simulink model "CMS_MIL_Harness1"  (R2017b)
settings: Solver=FixedStepDiscrete  StartTime=0.0  StopTime=23  FixedStep=0.01  RelTol=1e-3  EnableMultiTasking=on
undefined symbols (not defined in the file): sigbuilder_block
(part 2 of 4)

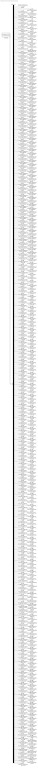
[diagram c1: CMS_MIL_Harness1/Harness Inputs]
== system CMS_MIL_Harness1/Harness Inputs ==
  Demux : Demux  Tag=STV Demux  Outputs=413
  FromWs : FromWorkspace  Tag=STV FromWs  VariableName=tuvar  SampleTime=0
  GeCTC_CtrCtlState_enum : Outport  Tag=STV Outport
  GbCTC_NegCtlState_flg : Outport  Tag=STV Outport  Port=2
  GbCTC_PosCtlState_flg : Outport  Tag=STV Outport  Port=3
  GbCTC_DCPosChrgCtlState_flg : Outport  Tag=STV Outport  Port=4
  GbCTC_DCNegChrgCtlState_flg : Outport  Tag=STV Outport  Port=5
  GcHDP_PackVolt_V : Outport  Tag=STV Outport  Port=6
  GbCTC_PreChrgCtlState_flg : Outport  Tag=STV Outport  Port=7
  GcHDP_PackCrnt_A : Outport  Tag=STV Outport  Port=8
  GbWSM_Kl15WkUpPrs_flg : Outport  Tag=STV Outport  Port=9
  GcCDP_MinCellVolt_mV : Outport  Tag=STV Outport  Port=10
  GcCDP_MaxCellVolt_mV : Outport  Tag=STV Outport  Port=11
  GbACC_ObcChrgCmd_flg : Outport  Tag=STV Outport  Port=12
  GcACC_ACChrgVoltRqst_V : Outport  Tag=STV Outport  Port=13
  GcACC_ACChrgCrntRqst_A : Outport  Tag=STV Outport  Port=14
  GbACC_ACChrgRqst_flg : Outport  Tag=STV Outport  Port=15
  GeCTC_CtrCtlConnMode_enum : Outport  Tag=STV Outport  Port=16
  GbMSM_SelfCheck_flg : Outport  Tag=STV Outport  Port=17
  GcSOC_DispSOC_pct : Outport  Tag=STV Outport  Port=18
  GbISP_TFHvilLFlt_flg : Outport  Tag=STV Outport  Port=19
  GeFTC_FltLvlOnCAN_enum : Outport  Tag=STV Outport  Port=20
  GcSOH_PackSOH_pct : Outport  Tag=STV Outport  Port=21
  GcSOC_PackSOC_pct : Outport  Tag=STV Outport  Port=22
  GcHDP_HallCrnt_A : Outport  Tag=STV Outport  Port=23
  GbMSM_SelfChckMaxTiReach_flg : Outport  Tag=STV Outport  Port=24
  GaCBC_CellBalCtlCmd_flg(1) : Outport  Tag=STV Outport  Port=25
  GaCBC_CellBalCtlCmd_flg(2) : Outport  Tag=STV Outport  Port=26
  GaCBC_CellBalCtlCmd_flg(3) : Outport  Tag=STV Outport  Port=27
  GaCBC_CellBalCtlCmd_flg(4) : Outport  Tag=STV Outport  Port=28
  GaCBC_CellBalCtlCmd_flg(5) : Outport  Tag=STV Outport  Port=29
  GaCBC_CellBalCtlCmd_flg(6) : Outport  Tag=STV Outport  Port=30
  GaCBC_CellBalCtlCmd_flg(7) : Outport  Tag=STV Outport  Port=31
  GaCBC_CellBalCtlCmd_flg(8) : Outport  Tag=STV Outport  Port=32
  GaCBC_CellBalCtlCmd_flg(9) : Outport  Tag=STV Outport  Port=33
  GaCBC_CellBalCtlCmd_flg(10) : Outport  Tag=STV Outport  Port=34
  GaCBC_CellBalCtlCmd_flg(11) : Outport  Tag=STV Outport  Port=35
  GaCBC_CellBalCtlCmd_flg(12) : Outport  Tag=STV Outport  Port=36
  GaCBC_CellBalCtlCmd_flg(13) : Outport  Tag=STV Outport  Port=37
  GaCBC_CellBalCtlCmd_flg(14) : Outport  Tag=STV Outport  Port=38
  GaCBC_CellBalCtlCmd_flg(15) : Outport  Tag=STV Outport  Port=39
  GaCBC_CellBalCtlCmd_flg(16) : Outport  Tag=STV Outport  Port=40
  GaCBC_CellBalCtlCmd_flg(17) : Outport  Tag=STV Outport  Port=41
  GaCBC_CellBalCtlCmd_flg(18) : Outport  Tag=STV Outport  Port=42
  GaCBC_CellBalCtlCmd_flg(19) : Outport  Tag=STV Outport  Port=43
  GaCBC_CellBalCtlCmd_flg(20) : Outport  Tag=STV Outport  Port=44
  GaCBC_CellBalCtlCmd_flg(21) : Outport  Tag=STV Outport  Port=45
  GaCBC_CellBalCtlCmd_flg(22) : Outport  Tag=STV Outport  Port=46
  GaCBC_CellBalCtlCmd_flg(23) : Outport  Tag=STV Outport  Port=47
  GaCBC_CellBalCtlCmd_flg(24) : Outport  Tag=STV Outport  Port=48
  GaCBC_CellBalCtlCmd_flg(25) : Outport  Tag=STV Outport  Port=49
  GaCBC_CellBalCtlCmd_flg(26) : Outport  Tag=STV Outport  Port=50
  GaCBC_CellBalCtlCmd_flg(27) : Outport  Tag=STV Outport  Port=51
  GaCBC_CellBalCtlCmd_flg(28) : Outport  Tag=STV Outport  Port=52
  GaCBC_CellBalCtlCmd_flg(29) : Outport  Tag=STV Outport  Port=53
  GaCBC_CellBalCtlCmd_flg(30) : Outport  Tag=STV Outport  Port=54
  GaCBC_CellBalCtlCmd_flg(31) : Outport  Tag=STV Outport  Port=55
  GaCBC_CellBalCtlCmd_flg(32) : Outport  Tag=STV Outport  Port=56
  GaCBC_CellBalCtlCmd_flg(33) : Outport  Tag=STV Outport  Port=57
  GaCBC_CellBalCtlCmd_flg(34) : Outport  Tag=STV Outport  Port=58
  GaCBC_CellBalCtlCmd_flg(35) : Outport  Tag=STV Outport  Port=59
  GaCBC_CellBalCtlCmd_flg(36) : Outport  Tag=STV Outport  Port=60
  GaCBC_CellBalCtlCmd_flg(37) : Outport  Tag=STV Outport  Port=61
  GaCBC_CellBalCtlCmd_flg(38) : Outport  Tag=STV Outport  Port=62
  GaCBC_CellBalCtlCmd_flg(39) : Outport  Tag=STV Outport  Port=63
  GaCBC_CellBalCtlCmd_flg(40) : Outport  Tag=STV Outport  Port=64
  GaCBC_CellBalCtlCmd_flg(41) : Outport  Tag=STV Outport  Port=65
  GaCBC_CellBalCtlCmd_flg(42) : Outport  Tag=STV Outport  Port=66
  GaCBC_CellBalCtlCmd_flg(43) : Outport  Tag=STV Outport  Port=67
  GaCBC_CellBalCtlCmd_flg(44) : Outport  Tag=STV Outport  Port=68
  GaCBC_CellBalCtlCmd_flg(45) : Outport  Tag=STV Outport  Port=69
  GaCBC_CellBalCtlCmd_flg(46) : Outport  Tag=STV Outport  Port=70
  GaCBC_CellBalCtlCmd_flg(47) : Outport  Tag=STV Outport  Port=71
  GaCBC_CellBalCtlCmd_flg(48) : Outport  Tag=STV Outport  Port=72
  GaCBC_CellBalCtlCmd_flg(49) : Outport  Tag=STV Outport  Port=73
  GaCBC_CellBalCtlCmd_flg(50) : Outport  Tag=STV Outport  Port=74
  GaCBC_CellBalCtlCmd_flg(51) : Outport  Tag=STV Outport  Port=75
  GaCBC_CellBalCtlCmd_flg(52) : Outport  Tag=STV Outport  Port=76
  GaCBC_CellBalCtlCmd_flg(53) : Outport  Tag=STV Outport  Port=77
  GaCBC_CellBalCtlCmd_flg(54) : Outport  Tag=STV Outport  Port=78
  GaCBC_CellBalCtlCmd_flg(55) : Outport  Tag=STV Outport  Port=79
  GaCBC_CellBalCtlCmd_flg(56) : Outport  Tag=STV Outport  Port=80
  GaCBC_CellBalCtlCmd_flg(57) : Outport  Tag=STV Outport  Port=81
  GaCBC_CellBalCtlCmd_flg(58) : Outport  Tag=STV Outport  Port=82
  GaCBC_CellBalCtlCmd_flg(59) : Outport  Tag=STV Outport  Port=83
  GaCBC_CellBalCtlCmd_flg(60) : Outport  Tag=STV Outport  Port=84
  GaCBC_CellBalCtlCmd_flg(61) : Outport  Tag=STV Outport  Port=85
  GaCBC_CellBalCtlCmd_flg(62) : Outport  Tag=STV Outport  Port=86
  GaCBC_CellBalCtlCmd_flg(63) : Outport  Tag=STV Outport  Port=87
  GaCBC_CellBalCtlCmd_flg(64) : Outport  Tag=STV Outport  Port=88
  GaCBC_CellBalCtlCmd_flg(65) : Outport  Tag=STV Outport  Port=89
  GaCBC_CellBalCtlCmd_flg(66) : Outport  Tag=STV Outport  Port=90
  GaCBC_CellBalCtlCmd_flg(67) : Outport  Tag=STV Outport  Port=91
  GaCBC_CellBalCtlCmd_flg(68) : Outport  Tag=STV Outport  Port=92
  GaCBC_CellBalCtlCmd_flg(69) : Outport  Tag=STV Outport  Port=93
  GaCBC_CellBalCtlCmd_flg(70) : Outport  Tag=STV Outport  Port=94
  GaCBC_CellBalCtlCmd_flg(71) : Outport  Tag=STV Outport  Port=95
  GaCBC_CellBalCtlCmd_flg(72) : Outport  Tag=STV Outport  Port=96
  GaCBC_CellBalCtlCmd_flg(73) : Outport  Tag=STV Outport  Port=97
  GaCBC_CellBalCtlCmd_flg(74) : Outport  Tag=STV Outport  Port=98
  GaCBC_CellBalCtlCmd_flg(75) : Outport  Tag=STV Outport  Port=99
  GaCBC_CellBalCtlCmd_flg(76) : Outport  Tag=STV Outport  Port=100
  GaCBC_CellBalCtlCmd_flg(77) : Outport  Tag=STV Outport  Port=101
  GaCBC_CellBalCtlCmd_flg(78) : Outport  Tag=STV Outport  Port=102
  GaCBC_CellBalCtlCmd_flg(79) : Outport  Tag=STV Outport  Port=103
  GaCBC_CellBalCtlCmd_flg(80) : Outport  Tag=STV Outport  Port=104
  GaCBC_CellBalCtlCmd_flg(81) : Outport  Tag=STV Outport  Port=105
  GaCBC_CellBalCtlCmd_flg(82) : Outport  Tag=STV Outport  Port=106
  GaCBC_CellBalCtlCmd_flg(83) : Outport  Tag=STV Outport  Port=107
  GaCBC_CellBalCtlCmd_flg(84) : Outport  Tag=STV Outport  Port=108
  GaCBC_CellBalCtlCmd_flg(85) : Outport  Tag=STV Outport  Port=109
  GaCBC_CellBalCtlCmd_flg(86) : Outport  Tag=STV Outport  Port=110
  GaCBC_CellBalCtlCmd_flg(87) : Outport  Tag=STV Outport  Port=111
  GaCBC_CellBalCtlCmd_flg(88) : Outport  Tag=STV Outport  Port=112
  GaCBC_CellBalCtlCmd_flg(89) : Outport  Tag=STV Outport  Port=113
  GaCBC_CellBalCtlCmd_flg(90) : Outport  Tag=STV Outport  Port=114
  GaCBC_CellBalCtlCmd_flg(91) : Outport  Tag=STV Outport  Port=115
  GaCBC_CellBalCtlCmd_flg(92) : Outport  Tag=STV Outport  Port=116
  GaCBC_CellBalCtlCmd_flg(93) : Outport  Tag=STV Outport  Port=117
  GaCBC_CellBalCtlCmd_flg(94) : Outport  Tag=STV Outport  Port=118
  GaCBC_CellBalCtlCmd_flg(95) : Outport  Tag=STV Outport  Port=119
  GaCBC_CellBalCtlCmd_flg(96) : Outport  Tag=STV Outport  Port=120
  GaCBC_CellBalCtlCmd_flg(97) : Outport  Tag=STV Outport  Port=121
  GaCBC_CellBalCtlCmd_flg(98) : Outport  Tag=STV Outport  Port=122
  GaCBC_CellBalCtlCmd_flg(99) : Outport  Tag=STV Outport  Port=123
  GaCBC_CellBalCtlCmd_flg(100) : Outport  Tag=STV Outport  Port=124
  GaCBC_CellBalCtlCmd_flg(101) : Outport  Tag=STV Outport  Port=125
  GaCBC_CellBalCtlCmd_flg(102) : Outport  Tag=STV Outport  Port=126
  GaCBC_CellBalCtlCmd_flg(103) : Outport  Tag=STV Outport  Port=127
  GaCBC_CellBalCtlCmd_flg(104) : Outport  Tag=STV Outport  Port=128
  GaCBC_CellBalCtlCmd_flg(105) : Outport  Tag=STV Outport  Port=129
  GaCBC_CellBalCtlCmd_flg(106) : Outport  Tag=STV Outport  Port=130
  GaCBC_CellBalCtlCmd_flg(107) : Outport  Tag=STV Outport  Port=131
  GaCBC_CellBalCtlCmd_flg(108) : Outport  Tag=STV Outport  Port=132
  GaCBC_CellBalCtlCmd_flg(109) : Outport  Tag=STV Outport  Port=133
  GaCBC_CellBalCtlCmd_flg(110) : Outport  Tag=STV Outport  Port=134
  GaCBC_CellBalCtlCmd_flg(111) : Outport  Tag=STV Outport  Port=135
  GaCBC_CellBalCtlCmd_flg(112) : Outport  Tag=STV Outport  Port=136
  GbDCC_DCChrgRqst_flg : Outport  Tag=STV Outport  Port=137
  GcSOP_DischrgConstPwr_kW : Outport  Tag=STV Outport  Port=138
  GcSOP_ChrgConstPwr_kW : Outport  Tag=STV Outport  Port=139
  GcISO_HVIsoValue_kohm : Outport  Tag=STV Outport  Port=140
  GeODP_ObcCcSt_enum : Outport  Tag=STV Outport  Port=141
  GbDCC_DCChrgFinish_flg : Outport  Tag=STV Outport  Port=142
  GbACC_ACChrgFinish_flg : Outport  Tag=STV Outport  Port=143
  GeACC_ACChrgState_enum : Outport  Tag=STV Outport  Port=144
  GeDCC_DCConnSt_enum : Outport  Tag=STV Outport  Port=145
  GeLDP_CC2St_enum : Outport  Tag=STV Outport  Port=146
  GcCDP_AvgCellTemp_C : Outport  Tag=STV Outport  Port=147
  GbISO_IsoForbid_flg : Outport  Tag=STV Outport  Port=148
  GcCDP_MaxCellTemp_C : Outport  Tag=STV Outport  Port=149
  GcCDP_MinCellTemp_C : Outport  Tag=STV Outport  Port=150
  GcDCS_3072ChrgVoltReq_V : Outport  Tag=STV Outport  Port=151
  GcDCC_DCChrgCrntRqst_A : Outport  Tag=STV Outport  Port=152
  GaCDP_CellVolt_mV(1) : Outport  Tag=STV Outport  Port=153
  GaCDP_CellVolt_mV(2) : Outport  Tag=STV Outport  Port=154
  GaCDP_CellVolt_mV(3) : Outport  Tag=STV Outport  Port=155
  GaCDP_CellVolt_mV(4) : Outport  Tag=STV Outport  Port=156
  GaCDP_CellVolt_mV(5) : Outport  Tag=STV Outport  Port=157
  GaCDP_CellVolt_mV(6) : Outport  Tag=STV Outport  Port=158
  GaCDP_CellVolt_mV(7) : Outport  Tag=STV Outport  Port=159
  GaCDP_CellVolt_mV(8) : Outport  Tag=STV Outport  Port=160
  GaCDP_CellVolt_mV(9) : Outport  Tag=STV Outport  Port=161
  GaCDP_CellVolt_mV(10) : Outport  Tag=STV Outport  Port=162
  GaCDP_CellVolt_mV(11) : Outport  Tag=STV Outport  Port=163
  GaCDP_CellVolt_mV(12) : Outport  Tag=STV Outport  Port=164
  GaCDP_CellVolt_mV(13) : Outport  Tag=STV Outport  Port=165
  GaCDP_CellVolt_mV(14) : Outport  Tag=STV Outport  Port=166
  GaCDP_CellVolt_mV(15) : Outport  Tag=STV Outport  Port=167
  GaCDP_CellVolt_mV(16) : Outport  Tag=STV Outport  Port=168
  GaCDP_CellVolt_mV(17) : Outport  Tag=STV Outport  Port=169
  GaCDP_CellVolt_mV(18) : Outport  Tag=STV Outport  Port=170
  GaCDP_CellVolt_mV(19) : Outport  Tag=STV Outport  Port=171
  GaCDP_CellVolt_mV(20) : Outport  Tag=STV Outport  Port=172
  GaCDP_CellVolt_mV(21) : Outport  Tag=STV Outport  Port=173
  GaCDP_CellVolt_mV(22) : Outport  Tag=STV Outport  Port=174
  GaCDP_CellVolt_mV(23) : Outport  Tag=STV Outport  Port=175
  GaCDP_CellVolt_mV(24) : Outport  Tag=STV Outport  Port=176
  GaCDP_CellVolt_mV(25) : Outport  Tag=STV Outport  Port=177
  GaCDP_CellVolt_mV(26) : Outport  Tag=STV Outport  Port=178
  GaCDP_CellVolt_mV(27) : Outport  Tag=STV Outport  Port=179
  GaCDP_CellVolt_mV(28) : Outport  Tag=STV Outport  Port=180
  GaCDP_CellVolt_mV(29) : Outport  Tag=STV Outport  Port=181
  GaCDP_CellVolt_mV(30) : Outport  Tag=STV Outport  Port=182
  GaCDP_CellVolt_mV(31) : Outport  Tag=STV Outport  Port=183
  GaCDP_CellVolt_mV(32) : Outport  Tag=STV Outport  Port=184
  GaCDP_CellVolt_mV(33) : Outport  Tag=STV Outport  Port=185
  GaCDP_CellVolt_mV(34) : Outport  Tag=STV Outport  Port=186
  GaCDP_CellVolt_mV(35) : Outport  Tag=STV Outport  Port=187
  GaCDP_CellVolt_mV(36) : Outport  Tag=STV Outport  Port=188
  GaCDP_CellVolt_mV(37) : Outport  Tag=STV Outport  Port=189
  GaCDP_CellVolt_mV(38) : Outport  Tag=STV Outport  Port=190
  GaCDP_CellVolt_mV(39) : Outport  Tag=STV Outport  Port=191
  GaCDP_CellVolt_mV(40) : Outport  Tag=STV Outport  Port=192
  GaCDP_CellVolt_mV(41) : Outport  Tag=STV Outport  Port=193
  GaCDP_CellVolt_mV(42) : Outport  Tag=STV Outport  Port=194
  GaCDP_CellVolt_mV(43) : Outport  Tag=STV Outport  Port=195
  GaCDP_CellVolt_mV(44) : Outport  Tag=STV Outport  Port=196
  GaCDP_CellVolt_mV(45) : Outport  Tag=STV Outport  Port=197
  GaCDP_CellVolt_mV(46) : Outport  Tag=STV Outport  Port=198
  GaCDP_CellVolt_mV(47) : Outport  Tag=STV Outport  Port=199
  GaCDP_CellVolt_mV(48) : Outport  Tag=STV Outport  Port=200
  GaCDP_CellVolt_mV(49) : Outport  Tag=STV Outport  Port=201
  GaCDP_CellVolt_mV(50) : Outport  Tag=STV Outport  Port=202
  GaCDP_CellVolt_mV(51) : Outport  Tag=STV Outport  Port=203
  GaCDP_CellVolt_mV(52) : Outport  Tag=STV Outport  Port=204
  GaCDP_CellVolt_mV(53) : Outport  Tag=STV Outport  Port=205
  GaCDP_CellVolt_mV(54) : Outport  Tag=STV Outport  Port=206
  GaCDP_CellVolt_mV(55) : Outport  Tag=STV Outport  Port=207
  GaCDP_CellVolt_mV(56) : Outport  Tag=STV Outport  Port=208
  GaCDP_CellVolt_mV(57) : Outport  Tag=STV Outport  Port=209
  GaCDP_CellVolt_mV(58) : Outport  Tag=STV Outport  Port=210
  GaCDP_CellVolt_mV(59) : Outport  Tag=STV Outport  Port=211
  GaCDP_CellVolt_mV(60) : Outport  Tag=STV Outport  Port=212
  GaCDP_CellVolt_mV(61) : Outport  Tag=STV Outport  Port=213
  GaCDP_CellVolt_mV(62) : Outport  Tag=STV Outport  Port=214
  GaCDP_CellVolt_mV(63) : Outport  Tag=STV Outport  Port=215
  GaCDP_CellVolt_mV(64) : Outport  Tag=STV Outport  Port=216
  GaCDP_CellVolt_mV(65) : Outport  Tag=STV Outport  Port=217
  GaCDP_CellVolt_mV(66) : Outport  Tag=STV Outport  Port=218
  GaCDP_CellVolt_mV(67) : Outport  Tag=STV Outport  Port=219
  GaCDP_CellVolt_mV(68) : Outport  Tag=STV Outport  Port=220
  GaCDP_CellVolt_mV(69) : Outport  Tag=STV Outport  Port=221
  GaCDP_CellVolt_mV(70) : Outport  Tag=STV Outport  Port=222
  GaCDP_CellVolt_mV(71) : Outport  Tag=STV Outport  Port=223
  GaCDP_CellVolt_mV(72) : Outport  Tag=STV Outport  Port=224
  GaCDP_CellVolt_mV(73) : Outport  Tag=STV Outport  Port=225
  GaCDP_CellVolt_mV(74) : Outport  Tag=STV Outport  Port=226
  GaCDP_CellVolt_mV(75) : Outport  Tag=STV Outport  Port=227
  GaCDP_CellVolt_mV(76) : Outport  Tag=STV Outport  Port=228
  GaCDP_CellVolt_mV(77) : Outport  Tag=STV Outport  Port=229
  GaCDP_CellVolt_mV(78) : Outport  Tag=STV Outport  Port=230
  GaCDP_CellVolt_mV(79) : Outport  Tag=STV Outport  Port=231
  GaCDP_CellVolt_mV(80) : Outport  Tag=STV Outport  Port=232
  GaCDP_CellVolt_mV(81) : Outport  Tag=STV Outport  Port=233
  GaCDP_CellVolt_mV(82) : Outport  Tag=STV Outport  Port=234
  GaCDP_CellVolt_mV(83) : Outport  Tag=STV Outport  Port=235
  GaCDP_CellVolt_mV(84) : Outport  Tag=STV Outport  Port=236
  GaCDP_CellVolt_mV(85) : Outport  Tag=STV Outport  Port=237
  GaCDP_CellVolt_mV(86) : Outport  Tag=STV Outport  Port=238
  GaCDP_CellVolt_mV(87) : Outport  Tag=STV Outport  Port=239
  GaCDP_CellVolt_mV(88) : Outport  Tag=STV Outport  Port=240
  GaCDP_CellVolt_mV(89) : Outport  Tag=STV Outport  Port=241
  GaCDP_CellVolt_mV(90) : Outport  Tag=STV Outport  Port=242
  GaCDP_CellVolt_mV(91) : Outport  Tag=STV Outport  Port=243
  GaCDP_CellVolt_mV(92) : Outport  Tag=STV Outport  Port=244
  GaCDP_CellVolt_mV(93) : Outport  Tag=STV Outport  Port=245
  GaCDP_CellVolt_mV(94) : Outport  Tag=STV Outport  Port=246
  GaCDP_CellVolt_mV(95) : Outport  Tag=STV Outport  Port=247
  GaCDP_CellVolt_mV(96) : Outport  Tag=STV Outport  Port=248
  GaCDP_CellVolt_mV(97) : Outport  Tag=STV Outport  Port=249
  GaCDP_CellVolt_mV(98) : Outport  Tag=STV Outport  Port=250
  GaCDP_CellVolt_mV(99) : Outport  Tag=STV Outport  Port=251
  GaCDP_CellVolt_mV(100) : Outport  Tag=STV Outport  Port=252
  GaCDP_CellVolt_mV(101) : Outport  Tag=STV Outport  Port=253
  GaCDP_CellVolt_mV(102) : Outport  Tag=STV Outport  Port=254
  GaCDP_CellVolt_mV(103) : Outport  Tag=STV Outport  Port=255
  GaCDP_CellVolt_mV(104) : Outport  Tag=STV Outport  Port=256
  GaCDP_CellVolt_mV(105) : Outport  Tag=STV Outport  Port=257
  GaCDP_CellVolt_mV(106) : Outport  Tag=STV Outport  Port=258
  GaCDP_CellVolt_mV(107) : Outport  Tag=STV Outport  Port=259
  GaCDP_CellVolt_mV(108) : Outport  Tag=STV Outport  Port=260
  GaCDP_CellVolt_mV(109) : Outport  Tag=STV Outport  Port=261
  GaCDP_CellVolt_mV(110) : Outport  Tag=STV Outport  Port=262
  GaCDP_CellVolt_mV(111) : Outport  Tag=STV Outport  Port=263
  GaCDP_CellVolt_mV(112) : Outport  Tag=STV Outport  Port=264
  GaCDP_CellTemp_C(1) : Outport  Tag=STV Outport  Port=265
  GaCDP_CellTemp_C(2) : Outport  Tag=STV Outport  Port=266
  GaCDP_CellTemp_C(3) : Outport  Tag=STV Outport  Port=267
  GaCDP_CellTemp_C(4) : Outport  Tag=STV Outport  Port=268
  GaCDP_CellTemp_C(5) : Outport  Tag=STV Outport  Port=269
  GaCDP_CellTemp_C(6) : Outport  Tag=STV Outport  Port=270
  GaCDP_CellTemp_C(7) : Outport  Tag=STV Outport  Port=271
  GaCDP_CellTemp_C(8) : Outport  Tag=STV Outport  Port=272
  GaCDP_CellTemp_C(9) : Outport  Tag=STV Outport  Port=273
  GaCDP_CellTemp_C(10) : Outport  Tag=STV Outport  Port=274
  GaCDP_CellTemp_C(11) : Outport  Tag=STV Outport  Port=275
  GaCDP_CellTemp_C(12) : Outport  Tag=STV Outport  Port=276
  GaCDP_CellTemp_C(13) : Outport  Tag=STV Outport  Port=277
  GaCDP_CellTemp_C(14) : Outport  Tag=STV Outport  Port=278
  GaCDP_CellTemp_C(15) : Outport  Tag=STV Outport  Port=279
  GaCDP_CellTemp_C(16) : Outport  Tag=STV Outport  Port=280
  GaCDP_CellTemp_C(17) : Outport  Tag=STV Outport  Port=281
  GaCDP_CellTemp_C(18) : Outport  Tag=STV Outport  Port=282
  GaCDP_CellTemp_C(19) : Outport  Tag=STV Outport  Port=283
  GaCDP_CellTemp_C(20) : Outport  Tag=STV Outport  Port=284
  GaCDP_CellTemp_C(21) : Outport  Tag=STV Outport  Port=285
  GaCDP_CellTemp_C(22) : Outport  Tag=STV Outport  Port=286
  GaCDP_CellTemp_C(23) : Outport  Tag=STV Outport  Port=287
  GaCDP_CellTemp_C(24) : Outport  Tag=STV Outport  Port=288
  GaCDP_CellTemp_C(25) : Outport  Tag=STV Outport  Port=289
  GaCDP_CellTemp_C(26) : Outport  Tag=STV Outport  Port=290
  GaCDP_CellTemp_C(27) : Outport  Tag=STV Outport  Port=291
  GaCDP_CellTemp_C(28) : Outport  Tag=STV Outport  Port=292
  GaCDP_CellTemp_C(29) : Outport  Tag=STV Outport  Port=293
  GaCDP_CellTemp_C(30) : Outport  Tag=STV Outport  Port=294
  GaCDP_CellTemp_C(31) : Outport  Tag=STV Outport  Port=295
  GaCDP_CellTemp_C(32) : Outport  Tag=STV Outport  Port=296
  GaCDP_CellTemp_C(33) : Outport  Tag=STV Outport  Port=297
  GaCDP_CellTemp_C(34) : Outport  Tag=STV Outport  Port=298
  GaCDP_CellTemp_C(35) : Outport  Tag=STV Outport  Port=299
  GaCDP_CellTemp_C(36) : Outport  Tag=STV Outport  Port=300
  GaCDP_CellTemp_C(37) : Outport  Tag=STV Outport  Port=301
  GaCDP_CellTemp_C(38) : Outport  Tag=STV Outport  Port=302
  GaCDP_CellTemp_C(39) : Outport  Tag=STV Outport  Port=303
  GaCDP_CellTemp_C(40) : Outport  Tag=STV Outport  Port=304
  GaCDP_CellTemp_C(41) : Outport  Tag=STV Outport  Port=305
  GaCDP_CellTemp_C(42) : Outport  Tag=STV Outport  Port=306
  GaCDP_CellTemp_C(43) : Outport  Tag=STV Outport  Port=307
  GaCDP_CellTemp_C(44) : Outport  Tag=STV Outport  Port=308
  GaCDP_CellTemp_C(45) : Outport  Tag=STV Outport  Port=309
  GaCDP_CellTemp_C(46) : Outport  Tag=STV Outport  Port=310
  GaCDP_CellTemp_C(47) : Outport  Tag=STV Outport  Port=311
  GaCDP_CellTemp_C(48) : Outport  Tag=STV Outport  Port=312
  GcLDP_lntWtTemp_C : Outport  Tag=STV Outport  Port=313
  GcLDP_OutWtTemp_C : Outport  Tag=STV Outport  Port=314
  GcBTM_CoolPwrReq_W : Outport  Tag=STV Outport  Port=315
  GcBTM_HeatPwrReq_W : Outport  Tag=STV Outport  Port=316
  GeBTM_CoolReq_enum : Outport  Tag=STV Outport  Port=317
  GeBTM_HeatReq_enum : Outport  Tag=STV Outport  Port=318
  GbODP_V2XDischrgCmd_flg : Outport  Tag=STV Outport  Port=319
  GeMSM_BMUState_enum : Outport  Tag=STV Outport  Port=320
  GcHDP_FuseVolt_V : Outport  Tag=STV Outport  Port=321
  GbADP_DischgReq_flg : Outport  Tag=STV Outport  Port=322
  GcHDP_PosCtlVolt_V : Outport  Tag=STV Outport  Port=323
  GcCDP_MaxCellVoltNumb_numb : Outport  Tag=STV Outport  Port=324
  GcCDP_MinCellVoltNumb_numb : Outport  Tag=STV Outport  Port=325
  GcCDP_MaxCellTempNumb_numb : Outport  Tag=STV Outport  Port=326
  GcCDP_MinCellTempNumb_numb : Outport  Tag=STV Outport  Port=327
  GbWSM_DCWkUpPrs_flg : Outport  Tag=STV Outport  Port=328
  GbACC_PreThmObcChrgCmd_flg : Outport  Tag=STV Outport  Port=329
  GbACC_PreThmRqst_flg : Outport  Tag=STV Outport  Port=330
  GcACC_PreThmCrntRqst_A : Outport  Tag=STV Outport  Port=331
  GcACC_PreThmVoltRqst_V : Outport  Tag=STV Outport  Port=332
  GbACC_PreHeatPrmt_flg : Outport  Tag=STV Outport  Port=333
  GbFTC_PowerDown_flg : Outport  Tag=STV Outport  Port=334
  GcBTM_CoolTempReq_C : Outport  Tag=STV Outport  Port=335
  GcBTM_HeatTempReq_C : Outport  Tag=STV Outport  Port=336
  GcACC_ChrgingTiRem_min : Outport  Tag=STV Outport  Port=337
  GcDCC_ChrgingTiRem_min : Outport  Tag=STV Outport  Port=338
  GeVDP_PreThmEna_enum : Outport  Tag=STV Outport  Port=339
  GcSOP_DischrgPwr_kW : Outport  Tag=STV Outport  Port=340
  GcSOP_ChrgPwr_kW : Outport  Tag=STV Outport  Port=341
  GcCDP_MaxBusbarTemp_C : Outport  Tag=STV Outport  Port=342
  GcCDP_MinBusbarTemp_C : Outport  Tag=STV Outport  Port=343
  GeDCC_DCChrgState_enum : Outport  Tag=STV Outport  Port=344
  GeLDP_ChrgGunConnSt_enum : Outport  Tag=STV Outport  Port=345
  GbISP_TFThmRnwyfDet_flg : Outport  Tag=STV Outport  Port=346
  GaCDP_BusbarTemp_C(1) : Outport  Tag=STV Outport  Port=347
  GaCDP_BusbarTemp_C(2) : Outport  Tag=STV Outport  Port=348
  GaCDP_BusbarTemp_C(3) : Outport  Tag=STV Outport  Port=349
  GaCDP_BusbarTemp_C(4) : Outport  Tag=STV Outport  Port=350
  GaCDP_BusbarTemp_C(5) : Outport  Tag=STV Outport  Port=351
  GaCDP_BusbarTemp_C(6) : Outport  Tag=STV Outport  Port=352
  GaCDP_BusbarTemp_C(7) : Outport  Tag=STV Outport  Port=353
  GaCDP_BusbarTemp_C(8) : Outport  Tag=STV Outport  Port=354
  GaCDP_BusbarTemp_C(9) : Outport  Tag=STV Outport  Port=355
  GaCDP_BusbarTemp_C(10) : Outport  Tag=STV Outport  Port=356
  GaCDP_BusbarTemp_C(11) : Outport  Tag=STV Outport  Port=357
  GaCDP_BusbarTemp_C(12) : Outport  Tag=STV Outport  Port=358
  GaCDP_BusbarTemp_C(13) : Outport  Tag=STV Outport  Port=359
  GaCDP_BusbarTemp_C(14) : Outport  Tag=STV Outport  Port=360
  GaCDP_BusbarTemp_C(15) : Outport  Tag=STV Outport  Port=361
  GaCDP_BusbarTemp_C(16) : Outport  Tag=STV Outport  Port=362
  GaCDP_BusbarTemp_C(17) : Outport  Tag=STV Outport  Port=363
  GaCDP_BusbarTemp_C(18) : Outport  Tag=STV Outport  Port=364
  GaCDP_BusbarTemp_C(19) : Outport  Tag=STV Outport  Port=365
  GaCDP_BusbarTemp_C(20) : Outport  Tag=STV Outport  Port=366
  GaCDP_BusbarTemp_C(21) : Outport  Tag=STV Outport  Port=367
  GaCDP_BusbarTemp_C(22) : Outport  Tag=STV Outport  Port=368
  GaCDP_BusbarTemp_C(23) : Outport  Tag=STV Outport  Port=369
  GaCDP_BusbarTemp_C(24) : Outport  Tag=STV Outport  Port=370
  GaCDP_BusbarTemp_C(25) : Outport  Tag=STV Outport  Port=371
  GaCDP_BusbarTemp_C(26) : Outport  Tag=STV Outport  Port=372
  GaCDP_BusbarTemp_C(27) : Outport  Tag=STV Outport  Port=373
  GaCDP_BusbarTemp_C(28) : Outport  Tag=STV Outport  Port=374
  GaCDP_BusbarTemp_C(29) : Outport  Tag=STV Outport  Port=375
  GaCDP_BusbarTemp_C(30) : Outport  Tag=STV Outport  Port=376
  GaCDP_BusbarTemp_C(31) : Outport  Tag=STV Outport  Port=377
  GaCDP_BusbarTemp_C(32) : Outport  Tag=STV Outport  Port=378
  GaCDP_BusbarTemp_C(33) : Outport  Tag=STV Outport  Port=379
  GaCDP_BusbarTemp_C(34) : Outport  Tag=STV Outport  Port=380
  GaCDP_BusbarTemp_C(35) : Outport  Tag=STV Outport  Port=381
  GaCDP_BusbarTemp_C(36) : Outport  Tag=STV Outport  Port=382
  GaCDP_BusbarTemp_C(37) : Outport  Tag=STV Outport  Port=383
  GaCDP_BusbarTemp_C(38) : Outport  Tag=STV Outport  Port=384
  GaCDP_BusbarTemp_C(39) : Outport  Tag=STV Outport  Port=385
  GaCDP_BusbarTemp_C(40) : Outport  Tag=STV Outport  Port=386
  GaCDP_BusbarTemp_C(41) : Outport  Tag=STV Outport  Port=387
  GaCDP_BusbarTemp_C(42) : Outport  Tag=STV Outport  Port=388
  GaCDP_BusbarTemp_C(43) : Outport  Tag=STV Outport  Port=389
  GaCDP_BusbarTemp_C(44) : Outport  Tag=STV Outport  Port=390
  GaCDP_BusbarTemp_C(45) : Outport  Tag=STV Outport  Port=391
  GaCDP_BusbarTemp_C(46) : Outport  Tag=STV Outport  Port=392
  GaCDP_BusbarTemp_C(47) : Outport  Tag=STV Outport  Port=393
  GaCDP_BusbarTemp_C(48) : Outport  Tag=STV Outport  Port=394
  GcUDS_CellTempNumb_numb : Outport  Tag=STV Outport  Port=395
  GcUDS_BusbarTempNumb_numb : Outport  Tag=STV Outport  Port=396
  GcUDS_CellVoltNum_numb : Outport  Tag=STV Outport  Port=397
  GcUDS_BatEnergy_kWh : Outport  Tag=STV Outport  Port=398
  GbACC_HoldTempPrmt_flg : Outport  Tag=STV Outport  Port=399
  GbACC_HoldTempObcChrgCmd_flg : Outport  Tag=STV Outport  Port=400
  GcACC_HoldTempVoltRqst_V : Outport  Tag=STV Outport  Port=401
  GcACC_HoldTempCrntRqst_A : Outport  Tag=STV Outport  Port=402
  GbACC_HoldTempRqst_flg : Outport  Tag=STV Outport  Port=403
  GbISP_TFIsoResFltLevel2_flg : Outport  Tag=STV Outport  Port=404
  GbISP_TFIsoDCResFltLevel2_flg : Outport  Tag=STV Outport  Port=405
  GbISP_TFIsoHVoffResFltLevel2_flg : Outport  Tag=STV Outport  Port=406
  GbISP_TFIsoResFltLevel1_flg : Outport  Tag=STV Outport  Port=407
  GbISP_TFIsoDCResFltLevel1_flg : Outport  Tag=STV Outport  Port=408
  GbISP_TFIsoHVoffResFltLevel1_flg : Outport  Tag=STV Outport  Port=409
  GbADP_OTAmodeONReq_flg : Outport  Tag=STV Outport  Port=410
  GeUDS_AreaSel_enum : Outport  Tag=STV Outport  Port=411
  GeDCC_ElockReq_enum : Outport  Tag=STV Outport  Port=412
  GeTRA_ThmRnwySt_enum : Outport  Tag=STV Outport  Port=413
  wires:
  FromWs/1 -> Demux/1
  Demux/1 -> GeCTC_CtrCtlState_enum/1
  Demux/2 -> GbCTC_NegCtlState_flg/1
  Demux/3 -> GbCTC_PosCtlState_flg/1
  Demux/4 -> GbCTC_DCPosChrgCtlState_flg/1
  Demux/5 -> GbCTC_DCNegChrgCtlState_flg/1
  Demux/6 -> GcHDP_PackVolt_V/1
  Demux/7 -> GbCTC_PreChrgCtlState_flg/1
  Demux/8 -> GcHDP_PackCrnt_A/1
  Demux/9 -> GbWSM_Kl15WkUpPrs_flg/1
  Demux/10 -> GcCDP_MinCellVolt_mV/1
  Demux/11 -> GcCDP_MaxCellVolt_mV/1
  Demux/12 -> GbACC_ObcChrgCmd_flg/1
  Demux/13 -> GcACC_ACChrgVoltRqst_V/1
  Demux/14 -> GcACC_ACChrgCrntRqst_A/1
  Demux/15 -> GbACC_ACChrgRqst_flg/1
  Demux/16 -> GeCTC_CtrCtlConnMode_enum/1
  Demux/17 -> GbMSM_SelfCheck_flg/1
  Demux/18 -> GcSOC_DispSOC_pct/1
  Demux/19 -> GbISP_TFHvilLFlt_flg/1
  Demux/20 -> GeFTC_FltLvlOnCAN_enum/1
  Demux/21 -> GcSOH_PackSOH_pct/1
  Demux/22 -> GcSOC_PackSOC_pct/1
  Demux/23 -> GcHDP_HallCrnt_A/1
  Demux/24 -> GbMSM_SelfChckMaxTiReach_flg/1
  Demux/25 -> GaCBC_CellBalCtlCmd_flg(1)/1
  Demux/26 -> GaCBC_CellBalCtlCmd_flg(2)/1
  Demux/27 -> GaCBC_CellBalCtlCmd_flg(3)/1
  Demux/28 -> GaCBC_CellBalCtlCmd_flg(4)/1
  Demux/29 -> GaCBC_CellBalCtlCmd_flg(5)/1
  Demux/30 -> GaCBC_CellBalCtlCmd_flg(6)/1
  Demux/31 -> GaCBC_CellBalCtlCmd_flg(7)/1
  Demux/32 -> GaCBC_CellBalCtlCmd_flg(8)/1
  Demux/33 -> GaCBC_CellBalCtlCmd_flg(9)/1
  Demux/34 -> GaCBC_CellBalCtlCmd_flg(10)/1
  Demux/35 -> GaCBC_CellBalCtlCmd_flg(11)/1
  Demux/36 -> GaCBC_CellBalCtlCmd_flg(12)/1
  Demux/37 -> GaCBC_CellBalCtlCmd_flg(13)/1
  Demux/38 -> GaCBC_CellBalCtlCmd_flg(14)/1
  Demux/39 -> GaCBC_CellBalCtlCmd_flg(15)/1
  Demux/40 -> GaCBC_CellBalCtlCmd_flg(16)/1
  Demux/41 -> GaCBC_CellBalCtlCmd_flg(17)/1
  Demux/42 -> GaCBC_CellBalCtlCmd_flg(18)/1
  Demux/43 -> GaCBC_CellBalCtlCmd_flg(19)/1
  Demux/44 -> GaCBC_CellBalCtlCmd_flg(20)/1
  Demux/45 -> GaCBC_CellBalCtlCmd_flg(21)/1
  Demux/46 -> GaCBC_CellBalCtlCmd_flg(22)/1
  Demux/47 -> GaCBC_CellBalCtlCmd_flg(23)/1
  Demux/48 -> GaCBC_CellBalCtlCmd_flg(24)/1
  Demux/49 -> GaCBC_CellBalCtlCmd_flg(25)/1
  Demux/50 -> GaCBC_CellBalCtlCmd_flg(26)/1
  Demux/51 -> GaCBC_CellBalCtlCmd_flg(27)/1
  Demux/52 -> GaCBC_CellBalCtlCmd_flg(28)/1
  Demux/53 -> GaCBC_CellBalCtlCmd_flg(29)/1
  Demux/54 -> GaCBC_CellBalCtlCmd_flg(30)/1
  Demux/55 -> GaCBC_CellBalCtlCmd_flg(31)/1
  Demux/56 -> GaCBC_CellBalCtlCmd_flg(32)/1
  Demux/57 -> GaCBC_CellBalCtlCmd_flg(33)/1
  Demux/58 -> GaCBC_CellBalCtlCmd_flg(34)/1
  Demux/59 -> GaCBC_CellBalCtlCmd_flg(35)/1
  Demux/60 -> GaCBC_CellBalCtlCmd_flg(36)/1
  Demux/61 -> GaCBC_CellBalCtlCmd_flg(37)/1
  Demux/62 -> GaCBC_CellBalCtlCmd_flg(38)/1
  Demux/63 -> GaCBC_CellBalCtlCmd_flg(39)/1
  Demux/64 -> GaCBC_CellBalCtlCmd_flg(40)/1
  Demux/65 -> GaCBC_CellBalCtlCmd_flg(41)/1
  Demux/66 -> GaCBC_CellBalCtlCmd_flg(42)/1
  Demux/67 -> GaCBC_CellBalCtlCmd_flg(43)/1
  Demux/68 -> GaCBC_CellBalCtlCmd_flg(44)/1
  Demux/69 -> GaCBC_CellBalCtlCmd_flg(45)/1
  Demux/70 -> GaCBC_CellBalCtlCmd_flg(46)/1
  Demux/71 -> GaCBC_CellBalCtlCmd_flg(47)/1
  Demux/72 -> GaCBC_CellBalCtlCmd_flg(48)/1
  Demux/73 -> GaCBC_CellBalCtlCmd_flg(49)/1
  Demux/74 -> GaCBC_CellBalCtlCmd_flg(50)/1
  Demux/75 -> GaCBC_CellBalCtlCmd_flg(51)/1
  Demux/76 -> GaCBC_CellBalCtlCmd_flg(52)/1
  Demux/77 -> GaCBC_CellBalCtlCmd_flg(53)/1
  Demux/78 -> GaCBC_CellBalCtlCmd_flg(54)/1
  Demux/79 -> GaCBC_CellBalCtlCmd_flg(55)/1
  Demux/80 -> GaCBC_CellBalCtlCmd_flg(56)/1
  Demux/81 -> GaCBC_CellBalCtlCmd_flg(57)/1
  Demux/82 -> GaCBC_CellBalCtlCmd_flg(58)/1
  Demux/83 -> GaCBC_CellBalCtlCmd_flg(59)/1
  Demux/84 -> GaCBC_CellBalCtlCmd_flg(60)/1
  Demux/85 -> GaCBC_CellBalCtlCmd_flg(61)/1
  Demux/86 -> GaCBC_CellBalCtlCmd_flg(62)/1
  Demux/87 -> GaCBC_CellBalCtlCmd_flg(63)/1
  Demux/88 -> GaCBC_CellBalCtlCmd_flg(64)/1
  Demux/89 -> GaCBC_CellBalCtlCmd_flg(65)/1
  Demux/90 -> GaCBC_CellBalCtlCmd_flg(66)/1
  Demux/91 -> GaCBC_CellBalCtlCmd_flg(67)/1
  Demux/92 -> GaCBC_CellBalCtlCmd_flg(68)/1
  Demux/93 -> GaCBC_CellBalCtlCmd_flg(69)/1
  Demux/94 -> GaCBC_CellBalCtlCmd_flg(70)/1
  Demux/95 -> GaCBC_CellBalCtlCmd_flg(71)/1
  Demux/96 -> GaCBC_CellBalCtlCmd_flg(72)/1
  Demux/97 -> GaCBC_CellBalCtlCmd_flg(73)/1
  Demux/98 -> GaCBC_CellBalCtlCmd_flg(74)/1
  Demux/99 -> GaCBC_CellBalCtlCmd_flg(75)/1
  Demux/100 -> GaCBC_CellBalCtlCmd_flg(76)/1
  Demux/101 -> GaCBC_CellBalCtlCmd_flg(77)/1
  Demux/102 -> GaCBC_CellBalCtlCmd_flg(78)/1
  Demux/103 -> GaCBC_CellBalCtlCmd_flg(79)/1
  Demux/104 -> GaCBC_CellBalCtlCmd_flg(80)/1
  Demux/105 -> GaCBC_CellBalCtlCmd_flg(81)/1
  Demux/106 -> GaCBC_CellBalCtlCmd_flg(82)/1
  Demux/107 -> GaCBC_CellBalCtlCmd_flg(83)/1
  Demux/108 -> GaCBC_CellBalCtlCmd_flg(84)/1
  Demux/109 -> GaCBC_CellBalCtlCmd_flg(85)/1
  Demux/110 -> GaCBC_CellBalCtlCmd_flg(86)/1
  Demux/111 -> GaCBC_CellBalCtlCmd_flg(87)/1
  Demux/112 -> GaCBC_CellBalCtlCmd_flg(88)/1
  Demux/113 -> GaCBC_CellBalCtlCmd_flg(89)/1
  Demux/114 -> GaCBC_CellBalCtlCmd_flg(90)/1
  Demux/115 -> GaCBC_CellBalCtlCmd_flg(91)/1
  Demux/116 -> GaCBC_CellBalCtlCmd_flg(92)/1
  Demux/117 -> GaCBC_CellBalCtlCmd_flg(93)/1
  Demux/118 -> GaCBC_CellBalCtlCmd_flg(94)/1
  Demux/119 -> GaCBC_CellBalCtlCmd_flg(95)/1
  Demux/120 -> GaCBC_CellBalCtlCmd_flg(96)/1
  Demux/121 -> GaCBC_CellBalCtlCmd_flg(97)/1
  Demux/122 -> GaCBC_CellBalCtlCmd_flg(98)/1
  Demux/123 -> GaCBC_CellBalCtlCmd_flg(99)/1
  Demux/124 -> GaCBC_CellBalCtlCmd_flg(100)/1
  Demux/125 -> GaCBC_CellBalCtlCmd_flg(101)/1
  Demux/126 -> GaCBC_CellBalCtlCmd_flg(102)/1
  Demux/127 -> GaCBC_CellBalCtlCmd_flg(103)/1
  Demux/128 -> GaCBC_CellBalCtlCmd_flg(104)/1
  Demux/129 -> GaCBC_CellBalCtlCmd_flg(105)/1
  Demux/130 -> GaCBC_CellBalCtlCmd_flg(106)/1
  Demux/131 -> GaCBC_CellBalCtlCmd_flg(107)/1
  Demux/132 -> GaCBC_CellBalCtlCmd_flg(108)/1
  Demux/133 -> GaCBC_CellBalCtlCmd_flg(109)/1
  Demux/134 -> GaCBC_CellBalCtlCmd_flg(110)/1
  Demux/135 -> GaCBC_CellBalCtlCmd_flg(111)/1
  Demux/136 -> GaCBC_CellBalCtlCmd_flg(112)/1
  Demux/137 -> GbDCC_DCChrgRqst_flg/1
  Demux/138 -> GcSOP_DischrgConstPwr_kW/1
  Demux/139 -> GcSOP_ChrgConstPwr_kW/1
  Demux/140 -> GcISO_HVIsoValue_kohm/1
  Demux/141 -> GeODP_ObcCcSt_enum/1
  Demux/142 -> GbDCC_DCChrgFinish_flg/1
  Demux/143 -> GbACC_ACChrgFinish_flg/1
  Demux/144 -> GeACC_ACChrgState_enum/1
  Demux/145 -> GeDCC_DCConnSt_enum/1
  Demux/146 -> GeLDP_CC2St_enum/1
  Demux/147 -> GcCDP_AvgCellTemp_C/1
  Demux/148 -> GbISO_IsoForbid_flg/1
  Demux/149 -> GcCDP_MaxCellTemp_C/1
  Demux/150 -> GcCDP_MinCellTemp_C/1
  Demux/151 -> GcDCS_3072ChrgVoltReq_V/1
  Demux/152 -> GcDCC_DCChrgCrntRqst_A/1
  Demux/153 -> GaCDP_CellVolt_mV(1)/1
  Demux/154 -> GaCDP_CellVolt_mV(2)/1
  Demux/155 -> GaCDP_CellVolt_mV(3)/1
  Demux/156 -> GaCDP_CellVolt_mV(4)/1
  Demux/157 -> GaCDP_CellVolt_mV(5)/1
  Demux/158 -> GaCDP_CellVolt_mV(6)/1
  Demux/159 -> GaCDP_CellVolt_mV(7)/1
  Demux/160 -> GaCDP_CellVolt_mV(8)/1
  Demux/161 -> GaCDP_CellVolt_mV(9)/1
  Demux/162 -> GaCDP_CellVolt_mV(10)/1
  Demux/163 -> GaCDP_CellVolt_mV(11)/1
  Demux/164 -> GaCDP_CellVolt_mV(12)/1
  Demux/165 -> GaCDP_CellVolt_mV(13)/1
  Demux/166 -> GaCDP_CellVolt_mV(14)/1
  Demux/167 -> GaCDP_CellVolt_mV(15)/1
  Demux/168 -> GaCDP_CellVolt_mV(16)/1
  Demux/169 -> GaCDP_CellVolt_mV(17)/1
  Demux/170 -> GaCDP_CellVolt_mV(18)/1
  Demux/171 -> GaCDP_CellVolt_mV(19)/1
  Demux/172 -> GaCDP_CellVolt_mV(20)/1
  Demux/173 -> GaCDP_CellVolt_mV(21)/1
  Demux/174 -> GaCDP_CellVolt_mV(22)/1
  Demux/175 -> GaCDP_CellVolt_mV(23)/1
  Demux/176 -> GaCDP_CellVolt_mV(24)/1
  Demux/177 -> GaCDP_CellVolt_mV(25)/1
  Demux/178 -> GaCDP_CellVolt_mV(26)/1
  Demux/179 -> GaCDP_CellVolt_mV(27)/1
  Demux/180 -> GaCDP_CellVolt_mV(28)/1
  Demux/181 -> GaCDP_CellVolt_mV(29)/1
  Demux/182 -> GaCDP_CellVolt_mV(30)/1
  Demux/183 -> GaCDP_CellVolt_mV(31)/1
  Demux/184 -> GaCDP_CellVolt_mV(32)/1
  Demux/185 -> GaCDP_CellVolt_mV(33)/1
  Demux/186 -> GaCDP_CellVolt_mV(34)/1
  Demux/187 -> GaCDP_CellVolt_mV(35)/1
  Demux/188 -> GaCDP_CellVolt_mV(36)/1
  Demux/189 -> GaCDP_CellVolt_mV(37)/1
  Demux/190 -> GaCDP_CellVolt_mV(38)/1
  Demux/191 -> GaCDP_CellVolt_mV(39)/1
  Demux/192 -> GaCDP_CellVolt_mV(40)/1
  Demux/193 -> GaCDP_CellVolt_mV(41)/1
  Demux/194 -> GaCDP_CellVolt_mV(42)/1
  Demux/195 -> GaCDP_CellVolt_mV(43)/1
  Demux/196 -> GaCDP_CellVolt_mV(44)/1
  Demux/197 -> GaCDP_CellVolt_mV(45)/1
  Demux/198 -> GaCDP_CellVolt_mV(46)/1
  Demux/199 -> GaCDP_CellVolt_mV(47)/1
  Demux/200 -> GaCDP_CellVolt_mV(48)/1
  Demux/201 -> GaCDP_CellVolt_mV(49)/1
  Demux/202 -> GaCDP_CellVolt_mV(50)/1
  Demux/203 -> GaCDP_CellVolt_mV(51)/1
  Demux/204 -> GaCDP_CellVolt_mV(52)/1
  Demux/205 -> GaCDP_CellVolt_mV(53)/1
  Demux/206 -> GaCDP_CellVolt_mV(54)/1
  Demux/207 -> GaCDP_CellVolt_mV(55)/1
  Demux/208 -> GaCDP_CellVolt_mV(56)/1
  Demux/209 -> GaCDP_CellVolt_mV(57)/1
  Demux/210 -> GaCDP_CellVolt_mV(58)/1
  Demux/211 -> GaCDP_CellVolt_mV(59)/1
  Demux/212 -> GaCDP_CellVolt_mV(60)/1
  Demux/213 -> GaCDP_CellVolt_mV(61)/1
  Demux/214 -> GaCDP_CellVolt_mV(62)/1
  Demux/215 -> GaCDP_CellVolt_mV(63)/1
  Demux/216 -> GaCDP_CellVolt_mV(64)/1
  Demux/217 -> GaCDP_CellVolt_mV(65)/1
  Demux/218 -> GaCDP_CellVolt_mV(66)/1
  Demux/219 -> GaCDP_CellVolt_mV(67)/1
  Demux/220 -> GaCDP_CellVolt_mV(68)/1
  Demux/221 -> GaCDP_CellVolt_mV(69)/1
  Demux/222 -> GaCDP_CellVolt_mV(70)/1
  Demux/223 -> GaCDP_CellVolt_mV(71)/1
  Demux/224 -> GaCDP_CellVolt_mV(72)/1
  Demux/225 -> GaCDP_CellVolt_mV(73)/1
  Demux/226 -> GaCDP_CellVolt_mV(74)/1
  Demux/227 -> GaCDP_CellVolt_mV(75)/1
  Demux/228 -> GaCDP_CellVolt_mV(76)/1
  Demux/229 -> GaCDP_CellVolt_mV(77)/1
  Demux/230 -> GaCDP_CellVolt_mV(78)/1
  Demux/231 -> GaCDP_CellVolt_mV(79)/1
  Demux/232 -> GaCDP_CellVolt_mV(80)/1
  Demux/233 -> GaCDP_CellVolt_mV(81)/1
  Demux/234 -> GaCDP_CellVolt_mV(82)/1
  Demux/235 -> GaCDP_CellVolt_mV(83)/1
  Demux/236 -> GaCDP_CellVolt_mV(84)/1
  Demux/237 -> GaCDP_CellVolt_mV(85)/1
  Demux/238 -> GaCDP_CellVolt_mV(86)/1
  Demux/239 -> GaCDP_CellVolt_mV(87)/1
  Demux/240 -> GaCDP_CellVolt_mV(88)/1
  Demux/241 -> GaCDP_CellVolt_mV(89)/1
  Demux/242 -> GaCDP_CellVolt_mV(90)/1
  Demux/243 -> GaCDP_CellVolt_mV(91)/1
  Demux/244 -> GaCDP_CellVolt_mV(92)/1
  Demux/245 -> GaCDP_CellVolt_mV(93)/1
  Demux/246 -> GaCDP_CellVolt_mV(94)/1
  Demux/247 -> GaCDP_CellVolt_mV(95)/1
  Demux/248 -> GaCDP_CellVolt_mV(96)/1
  Demux/249 -> GaCDP_CellVolt_mV(97)/1
  Demux/250 -> GaCDP_CellVolt_mV(98)/1
  Demux/251 -> GaCDP_CellVolt_mV(99)/1
  Demux/252 -> GaCDP_CellVolt_mV(100)/1
  Demux/253 -> GaCDP_CellVolt_mV(101)/1
  Demux/254 -> GaCDP_CellVolt_mV(102)/1
  Demux/255 -> GaCDP_CellVolt_mV(103)/1
  Demux/256 -> GaCDP_CellVolt_mV(104)/1
  Demux/257 -> GaCDP_CellVolt_mV(105)/1
  Demux/258 -> GaCDP_CellVolt_mV(106)/1
  Demux/259 -> GaCDP_CellVolt_mV(107)/1
  Demux/260 -> GaCDP_CellVolt_mV(108)/1
  Demux/261 -> GaCDP_CellVolt_mV(109)/1
  Demux/262 -> GaCDP_CellVolt_mV(110)/1
  Demux/263 -> GaCDP_CellVolt_mV(111)/1
  Demux/264 -> GaCDP_CellVolt_mV(112)/1
  Demux/265 -> GaCDP_CellTemp_C(1)/1
  Demux/266 -> GaCDP_CellTemp_C(2)/1
  Demux/267 -> GaCDP_CellTemp_C(3)/1
  Demux/268 -> GaCDP_CellTemp_C(4)/1
  Demux/269 -> GaCDP_CellTemp_C(5)/1
  Demux/270 -> GaCDP_CellTemp_C(6)/1
  Demux/271 -> GaCDP_CellTemp_C(7)/1
  Demux/272 -> GaCDP_CellTemp_C(8)/1
  Demux/273 -> GaCDP_CellTemp_C(9)/1
  Demux/274 -> GaCDP_CellTemp_C(10)/1
  Demux/275 -> GaCDP_CellTemp_C(11)/1
  Demux/276 -> GaCDP_CellTemp_C(12)/1
  Demux/277 -> GaCDP_CellTemp_C(13)/1
  Demux/278 -> GaCDP_CellTemp_C(14)/1
  Demux/279 -> GaCDP_CellTemp_C(15)/1
  Demux/280 -> GaCDP_CellTemp_C(16)/1
  Demux/281 -> GaCDP_CellTemp_C(17)/1
  Demux/282 -> GaCDP_CellTemp_C(18)/1
  Demux/283 -> GaCDP_CellTemp_C(19)/1
  Demux/284 -> GaCDP_CellTemp_C(20)/1
  Demux/285 -> GaCDP_CellTemp_C(21)/1
  Demux/286 -> GaCDP_CellTemp_C(22)/1
  Demux/287 -> GaCDP_CellTemp_C(23)/1
  Demux/288 -> GaCDP_CellTemp_C(24)/1
  Demux/289 -> GaCDP_CellTemp_C(25)/1
  Demux/290 -> GaCDP_CellTemp_C(26)/1
  Demux/291 -> GaCDP_CellTemp_C(27)/1
  Demux/292 -> GaCDP_CellTemp_C(28)/1
  Demux/293 -> GaCDP_CellTemp_C(29)/1
  Demux/294 -> GaCDP_CellTemp_C(30)/1
  Demux/295 -> GaCDP_CellTemp_C(31)/1
  Demux/296 -> GaCDP_CellTemp_C(32)/1
  Demux/297 -> GaCDP_CellTemp_C(33)/1
  Demux/298 -> GaCDP_CellTemp_C(34)/1
  Demux/299 -> GaCDP_CellTemp_C(35)/1
  Demux/300 -> GaCDP_CellTemp_C(36)/1
  Demux/301 -> GaCDP_CellTemp_C(37)/1
  Demux/302 -> GaCDP_CellTemp_C(38)/1
  Demux/303 -> GaCDP_CellTemp_C(39)/1
  Demux/304 -> GaCDP_CellTemp_C(40)/1
  Demux/305 -> GaCDP_CellTemp_C(41)/1
  Demux/306 -> GaCDP_CellTemp_C(42)/1
  Demux/307 -> GaCDP_CellTemp_C(43)/1
  Demux/308 -> GaCDP_CellTemp_C(44)/1
  Demux/309 -> GaCDP_CellTemp_C(45)/1
  Demux/310 -> GaCDP_CellTemp_C(46)/1
  Demux/311 -> GaCDP_CellTemp_C(47)/1
  Demux/312 -> GaCDP_CellTemp_C(48)/1
  Demux/313 -> GcLDP_lntWtTemp_C/1
  Demux/314 -> GcLDP_OutWtTemp_C/1
  Demux/315 -> GcBTM_CoolPwrReq_W/1
  Demux/316 -> GcBTM_HeatPwrReq_W/1
  Demux/317 -> GeBTM_CoolReq_enum/1
  Demux/318 -> GeBTM_HeatReq_enum/1
  Demux/319 -> GbODP_V2XDischrgCmd_flg/1
  Demux/320 -> GeMSM_BMUState_enum/1
  Demux/321 -> GcHDP_FuseVolt_V/1
  Demux/322 -> GbADP_DischgReq_flg/1
  Demux/323 -> GcHDP_PosCtlVolt_V/1
  Demux/324 -> GcCDP_MaxCellVoltNumb_numb/1
  Demux/325 -> GcCDP_MinCellVoltNumb_numb/1
  Demux/326 -> GcCDP_MaxCellTempNumb_numb/1
  Demux/327 -> GcCDP_MinCellTempNumb_numb/1
  Demux/328 -> GbWSM_DCWkUpPrs_flg/1
  Demux/329 -> GbACC_PreThmObcChrgCmd_flg/1
  Demux/330 -> GbACC_PreThmRqst_flg/1
  Demux/331 -> GcACC_PreThmCrntRqst_A/1
  Demux/332 -> GcACC_PreThmVoltRqst_V/1
  Demux/333 -> GbACC_PreHeatPrmt_flg/1
  Demux/334 -> GbFTC_PowerDown_flg/1
  Demux/335 -> GcBTM_CoolTempReq_C/1
  Demux/336 -> GcBTM_HeatTempReq_C/1
  Demux/337 -> GcACC_ChrgingTiRem_min/1
  Demux/338 -> GcDCC_ChrgingTiRem_min/1
  Demux/339 -> GeVDP_PreThmEna_enum/1
  Demux/340 -> GcSOP_DischrgPwr_kW/1
  Demux/341 -> GcSOP_ChrgPwr_kW/1
  Demux/342 -> GcCDP_MaxBusbarTemp_C/1
  Demux/343 -> GcCDP_MinBusbarTemp_C/1
  Demux/344 -> GeDCC_DCChrgState_enum/1
  Demux/345 -> GeLDP_ChrgGunConnSt_enum/1
  Demux/346 -> GbISP_TFThmRnwyfDet_flg/1
  Demux/347 -> GaCDP_BusbarTemp_C(1)/1
  Demux/348 -> GaCDP_BusbarTemp_C(2)/1
  Demux/349 -> GaCDP_BusbarTemp_C(3)/1
  Demux/350 -> GaCDP_BusbarTemp_C(4)/1
  Demux/351 -> GaCDP_BusbarTemp_C(5)/1
  Demux/352 -> GaCDP_BusbarTemp_C(6)/1
  Demux/353 -> GaCDP_BusbarTemp_C(7)/1
  Demux/354 -> GaCDP_BusbarTemp_C(8)/1
  Demux/355 -> GaCDP_BusbarTemp_C(9)/1
  Demux/356 -> GaCDP_BusbarTemp_C(10)/1
  Demux/357 -> GaCDP_BusbarTemp_C(11)/1
  Demux/358 -> GaCDP_BusbarTemp_C(12)/1
  Demux/359 -> GaCDP_BusbarTemp_C(13)/1
  Demux/360 -> GaCDP_BusbarTemp_C(14)/1
  Demux/361 -> GaCDP_BusbarTemp_C(15)/1
  Demux/362 -> GaCDP_BusbarTemp_C(16)/1
  Demux/363 -> GaCDP_BusbarTemp_C(17)/1
  Demux/364 -> GaCDP_BusbarTemp_C(18)/1
  Demux/365 -> GaCDP_BusbarTemp_C(19)/1
  Demux/366 -> GaCDP_BusbarTemp_C(20)/1
  Demux/367 -> GaCDP_BusbarTemp_C(21)/1
  Demux/368 -> GaCDP_BusbarTemp_C(22)/1
  Demux/369 -> GaCDP_BusbarTemp_C(23)/1
  Demux/370 -> GaCDP_BusbarTemp_C(24)/1
  Demux/371 -> GaCDP_BusbarTemp_C(25)/1
  Demux/372 -> GaCDP_BusbarTemp_C(26)/1
  Demux/373 -> GaCDP_BusbarTemp_C(27)/1
  Demux/374 -> GaCDP_BusbarTemp_C(28)/1
  Demux/375 -> GaCDP_BusbarTemp_C(29)/1
  Demux/376 -> GaCDP_BusbarTemp_C(30)/1
  Demux/377 -> GaCDP_BusbarTemp_C(31)/1
  Demux/378 -> GaCDP_BusbarTemp_C(32)/1
  Demux/379 -> GaCDP_BusbarTemp_C(33)/1
  Demux/380 -> GaCDP_BusbarTemp_C(34)/1
  Demux/381 -> GaCDP_BusbarTemp_C(35)/1
  Demux/382 -> GaCDP_BusbarTemp_C(36)/1
  Demux/383 -> GaCDP_BusbarTemp_C(37)/1
  Demux/384 -> GaCDP_BusbarTemp_C(38)/1
  Demux/385 -> GaCDP_BusbarTemp_C(39)/1
  Demux/386 -> GaCDP_BusbarTemp_C(40)/1
  Demux/387 -> GaCDP_BusbarTemp_C(41)/1
  Demux/388 -> GaCDP_BusbarTemp_C(42)/1
  Demux/389 -> GaCDP_BusbarTemp_C(43)/1
  Demux/390 -> GaCDP_BusbarTemp_C(44)/1
  Demux/391 -> GaCDP_BusbarTemp_C(45)/1
  Demux/392 -> GaCDP_BusbarTemp_C(46)/1
  Demux/393 -> GaCDP_BusbarTemp_C(47)/1
  Demux/394 -> GaCDP_BusbarTemp_C(48)/1
  Demux/395 -> GcUDS_CellTempNumb_numb/1
  Demux/396 -> GcUDS_BusbarTempNumb_numb/1
  Demux/397 -> GcUDS_CellVoltNum_numb/1
  Demux/398 -> GcUDS_BatEnergy_kWh/1
  Demux/399 -> GbACC_HoldTempPrmt_flg/1
  Demux/400 -> GbACC_HoldTempObcChrgCmd_flg/1
  Demux/401 -> GcACC_HoldTempVoltRqst_V/1
  Demux/402 -> GcACC_HoldTempCrntRqst_A/1
  Demux/403 -> GbACC_HoldTempRqst_flg/1
  Demux/404 -> GbISP_TFIsoResFltLevel2_flg/1
  Demux/405 -> GbISP_TFIsoDCResFltLevel2_flg/1
  Demux/406 -> GbISP_TFIsoHVoffResFltLevel2_flg/1
  Demux/407 -> GbISP_TFIsoResFltLevel1_flg/1
  Demux/408 -> GbISP_TFIsoDCResFltLevel1_flg/1
  Demux/409 -> GbISP_TFIsoHVoffResFltLevel1_flg/1
  Demux/410 -> GbADP_OTAmodeONReq_flg/1
  Demux/411 -> GeUDS_AreaSel_enum/1
  Demux/412 -> GeDCC_ElockReq_enum/1
  Demux/413 -> GeTRA_ThmRnwySt_enum/1
